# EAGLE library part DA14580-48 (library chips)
Dialog Semiconductor BLE chip
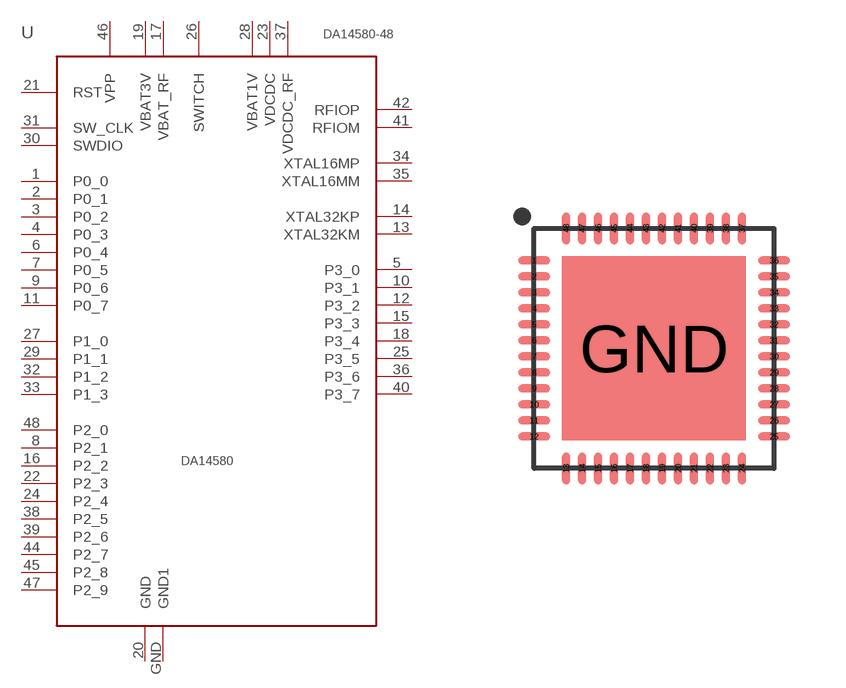
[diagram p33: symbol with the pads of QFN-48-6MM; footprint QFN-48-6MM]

Designator prefix U

## DA14580-48 (DIGIKEY: 1564-1014-1-ND)  [QFN-48-6MM]
1  P0_0
2  P0_1
3  P0_2
4  P0_3
5  P3_0
6  P0_4
7  P0_5
8  P2_1
9  P0_6
10  P3_1
11  P0_7
12  P3_2
13  XTAL32KM
14  XTAL32KP
15  P3_3
16  P2_2
17  VBAT_RF
18  P3_4
19  VBAT3V
20  GND
21  RST
22  P2_3
23  VDCDC
24  P2_4
25  P3_5
26  SWITCH
27  P1_0
28  VBAT1V
29  P1_1
30  SWDIO
31  SW_CLK
32  P1_2
33  P1_3
34  XTAL16MP
35  XTAL16MM
36  P3_6
37  VDCDC_RF
38  P2_5
39  P2_6
40  P3_7
41  RFIOM
42  RFIOP
44  P2_7
45  P2_8
46  VPP
47  P2_9
48  P2_0
GND  GND1

## Footprint QFN-48-6MM (pad centres in mm)
6MM x 6MM 48QFN package
smd 0.8 x 0.203: 1 -3,2.2; 2 -3,1.8; 3 -3,1.4; 4 -3,1; 5 -3,0.6; 6 -3,0.2; 7 -3,-0.2; 8 -3,-0.6; 9 -3,-1; 10 -3,-1.4; 11 -3,-1.8; 12 -3,-2.2; 25 3,-2.2; 26 3,-1.8; 27 3,-1.4; 28 3,-1; 29 3,-0.6; 30 3,-0.2; 31 3,0.2; 32 3,0.6; 33 3,1; 34 3,1.4; 35 3,1.8; 36 3,2.2
smd 0.203 x 0.8: 13 -2.2,-3; 14 -1.8,-3; 15 -1.4,-3; 16 -1,-3; 17 -0.6,-3; 18 -0.2,-3; 19 0.2,-3; 20 0.6,-3; 21 1,-3; 22 1.4,-3; 23 1.8,-3; 24 2.2,-3; 37 2.2,3; 38 1.8,3; 39 1.4,3; 40 1,3; 41 0.6,3; 42 0.2,3; 43 -0.2,3; 44 -0.6,3; 45 -1,3; 46 -1.4,3; 47 -1.8,3; 48 -2.2,3
smd 4.6 x 4.6: GND 0,0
